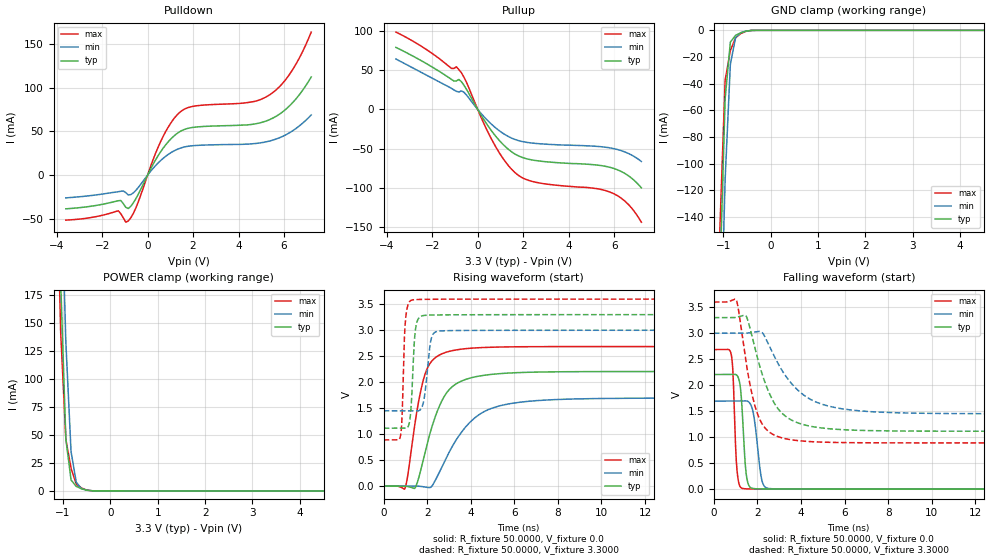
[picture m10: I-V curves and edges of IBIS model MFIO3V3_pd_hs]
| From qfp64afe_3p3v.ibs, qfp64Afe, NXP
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[Model] MFIO3V3_pd_hs
|   Model MFIO3V3_pd_hs
| This model was characterised for following simulation conditions:
| External (pad) voltage:
|   - Typ: 3.3V,   - Min: 3.0V,   - Max: 3.6V
| Library cells for typ/min/max conditions are connected as defined below:
|  IO - External Pad
|  A - Core Input
|  EN - Output Buffer Enable
|  BOOST - vdde
|  EHS - vdd
|  ENZI - vdd
|  EPD - vdd
|  EPUN - vdd
|  ZI - NC
|  ZIF - NC
|  gnd - gnd
|  gnde - gnde
|  vdd - vdd
|  vdde - vdde
| All other pins connected to ground
Model_type I/O
Polarity   Non-Inverting
Enable   Active-Low
Vinl =   0.9900V
Vinh =   2.3100V
Vmeas =  1.6500V
Cref =   0.0F
Rref =   100.0000
Vref =   0.0V
C_comp   1.5343pF   1.4580pF   1.6019pF
|C_comp_pullup   0.7283pF   0.7532pF   0.6914pF
|C_comp_pulldown   0.5932pF   0.6316pF   0.5575pF
[Model Spec]
| variable   typ   min   max
Vinh   0.9900V   0.9000V   1.0800V
Vinl   2.3100V   2.1000V   2.5200V
Vmeas   1.6500V   1.5000V   1.8000V
[Temperature Range]   25.0000   0.1250k   -40.0000
[Voltage Range]   3.3000V   3.0000V   3.6000V
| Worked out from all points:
|   slope of the pulldown table from 0 to 0.495 V, typ, clamps not added: 21 ohm
|   slope of the pullup table from 0 to 0.495 V, typ, clamps not added: 21.7 ohm
|   GND clamp passes 1 mA (typ) near -0.56 V on its own axis
|   POWER clamp passes 1 mA (typ) near -0.53 V on its own axis
|   rising waveform, R_fixture 50.0000, V_fixture 0.0: 20-80 % time 1.06ns typ, 1.67ns min, 677ps max; typ from 0 V to 2.21 V
|   rising waveform, R_fixture 50.0000, V_fixture 3.3000: 20-80 % time 158ps typ, 235ps min, 124ps max; typ from 1.11 V to 3.3 V
|   falling waveform, R_fixture 50.0000, V_fixture 0.0: 20-80 % time 188ps typ, 278ps min, 145ps max; typ from 2.21 V to 0 V
|   falling waveform, R_fixture 50.0000, V_fixture 3.3000: 20-80 % time 1.14ns typ, 1.68ns min, 748ps max; typ from 3.3 V to 1.11 V
[Pulldown]
|Voltage   I(typ)   I(min)   I(max)
-3.6V     -38.54mA   -26.03mA   -51.47mA
-1.29V    -29.27mA   -18.96mA   -40.78mA
-960mV    -36.81mA   -20.01mA   -53.83mA
-850mV    -38.18mA   -22.68mA   -52.4mA
-520mV    -27.12mA   -17.5mA    -37.74mA
580mV     26.98mA    16.83mA    38.78mA
1.35V     48.62mA    30.01mA    70.27mA
2.01V     54.62mA    33.69mA    78.71mA
4.43V     57.57mA    35.54mA    83.11mA
5.31V     62.85mA    38.64mA    90.87mA
6.3V      80.67mA    49.35mA    117.4mA
7.2V      112.3mA    68.85mA    163.6mA
[Pullup]
|Voltage   I(typ)   I(min)   I(max)
-3.6V     79.43mA    64.59mA    99.03mA
-1.05V    36.46mA    25.05mA    52.51mA
-830mV    38.41mA    22.29mA    50.98mA
-610mV    31.13mA    22.16mA    41.54mA
270mV     -13.03mA   -9.075mA   -18mA
710mV     -31.29mA   -21.6mA    -43.53mA
1.26V     -48.73mA   -33.16mA   -68.54mA
1.7V      -58.01mA   -38.97mA   -82.27mA
2.58V     -65.44mA   -43.49mA   -93.28mA
5.88V     -74.5mA    -49.46mA   -106.4mA
6.65V     -85.19mA   -56.54mA   -122.1mA
7.2V      -100.2mA   -66.51mA   -144.2mA
[GND_clamp]
|Voltage   I(typ)   I(min)   I(max)
-3.6V     -4.776A    -4.755A    -4.803A
-1.07V    -185.2mA   -255.8mA   -147.9mA
-960mV    -51.26mA   -111.8mA   -37.36mA
-850mV    -8.879mA   -25.45mA   -15.19mA
-740mV    -3.782mA   -5.531mA   -5.645mA
-630mV    -1.803mA   -1.784mA   -2.444mA
-520mV    -592.1uA   -582.6uA   -781uA
-300mV    -8.619uA   -12.3uA    -9.227uA
7.2V      0A         0A         0A
[POWER_clamp]
|Voltage   I(typ)   I(min)   I(max)
-3.6V     5.691A     5.665A     5.731A
-1.16V    387.4mA    485.6mA    339.3mA
-1.05V    187.9mA    295.9mA    142.8mA
-940mV    46.42mA    133mA      46.27mA
-830mV    9.779mA    35.03mA    20.21mA
-720mV    4.043mA    7.776mA    6.047mA
-610mV    1.916mA    2.078mA    2.613mA
-500mV    646.2uA    680.9uA    832.2uA
-280mV    73uA       65.71uA    91.35uA
7.2V      0A         0A         0A
[Ramp]
| variable   typ   min   max
dV/dt_r  1.3230/1.0595n   1.0165/1.6737n   1.6111/0.6768n
dV/dt_f  1.3109/1.1398n   0.9294/1.6804n   1.6255/0.7475n
R_load = 50.0000
[Rising Waveform]
R_fixture= 50.0000
V_fixture= 0.0
V_fixture_min= 0.0
V_fixture_max= 0.0
|time   V(typ)   V(min)   V(max)
0s        3.835nV    108.6nV    40.83nV
983.3ps   90.15uV    -26.54uV   -37.18mV
1.468ns   -16.76mV   257.5uV    1.288V
1.762ns   408.9mV    -8.567mV   1.944V
2.092ns   961.7mV    -29.03mV   2.337V
2.882ns   1.791V     549mV      2.578V
4.06ns    2.089V     1.268V     2.655V
5.815ns   2.177V     1.587V     2.68V
9.916ns   2.204V     1.686V     2.685V
100ns     2.205V     1.694V     2.685V
[Rising Waveform]
R_fixture= 50.0000
V_fixture= 3.3000
V_fixture_min= 3.0000
V_fixture_max= 3.6000
|time   V(typ)   V(min)   V(max)
0s        1.114V     1.45V      889.8mV
773.3ps   1.114V     1.45V      967.1mV
845ps     1.114V     1.45V      1.335V
976.6ps   1.113V     1.45V      3.047V
1.152ns   1.175V     1.45V      3.525V
1.452ns   2.986V     1.448V     3.588V
1.826ns   3.282V     1.614V     3.594V
2.211ns   3.292V     2.874V     3.596V
2.745ns   3.295V     2.989V     3.597V
100ns     3.299V     2.999V     3.599V
[Falling Waveform]
R_fixture= 50.0000
V_fixture= 0.0
V_fixture_min= 0.0
V_fixture_max= 0.0
|time   V(typ)   V(min)   V(max)
0s        2.205V     1.694V     2.685V
803ps     2.205V     1.694V     2.585V
875.3ps   2.206V     1.694V     2.28V
1.076ns   2.183V     1.694V     318.6mV
1.244ns   1.866V     1.694V     29.82mV
1.448ns   461.8mV    1.698V     6.954mV
1.804ns   12.9mV     1.484V     2.964mV
2.245ns   3.719mV    117mV      1.699mV
2.717ns   2.098mV    6.949mV    1.052mV
100ns     10.27nV    120nV      44.8nV
[Falling Waveform]
R_fixture= 50.0000
V_fixture= 3.3000
V_fixture_min= 3.0000
V_fixture_max= 3.6000
|time   V(typ)   V(min)   V(max)
0s        3.299V     2.999V     3.599V
1.047ns   3.307V     2.999V     3.627V
1.51ns    3.309V     3.001V     2.368V
1.858ns   2.766V     3.02V      1.645V
2.245ns   2.18V      3.001V     1.238V
3.053ns   1.495V     2.339V     995.6mV
4.328ns   1.22V      1.754V     917.3mV
6.45ns    1.134V     1.516V     893.8mV
10.6ns    1.115V     1.455V     889.9mV
100ns     1.114V     1.45V      889.8mV
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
